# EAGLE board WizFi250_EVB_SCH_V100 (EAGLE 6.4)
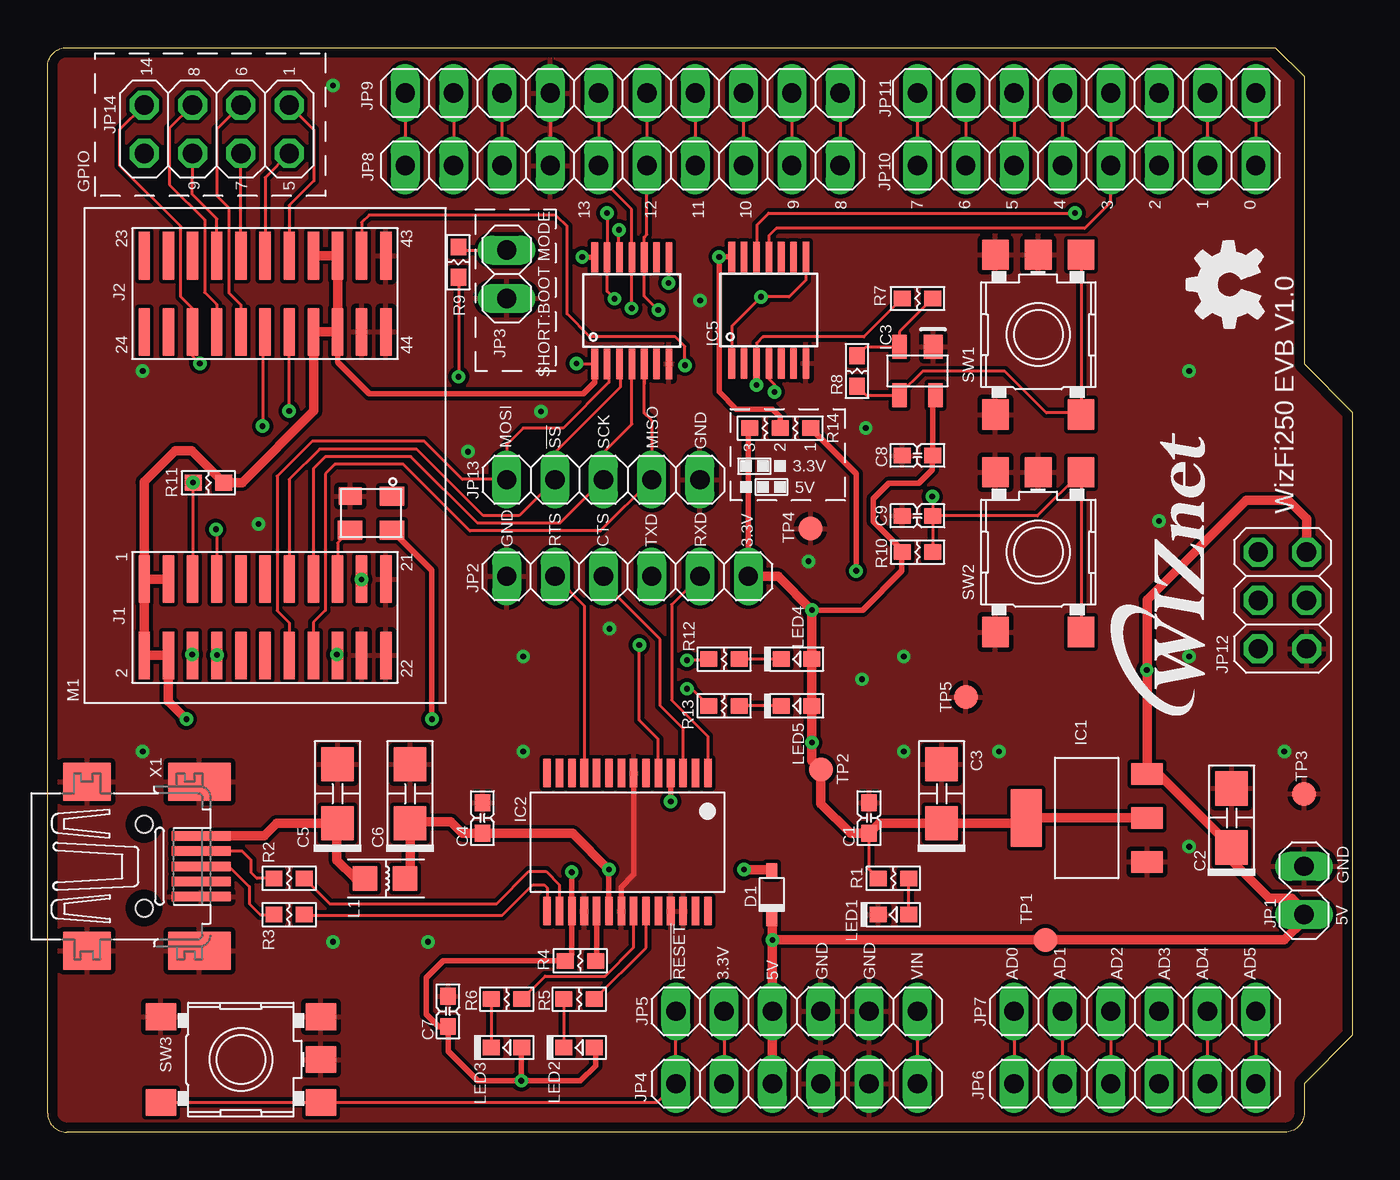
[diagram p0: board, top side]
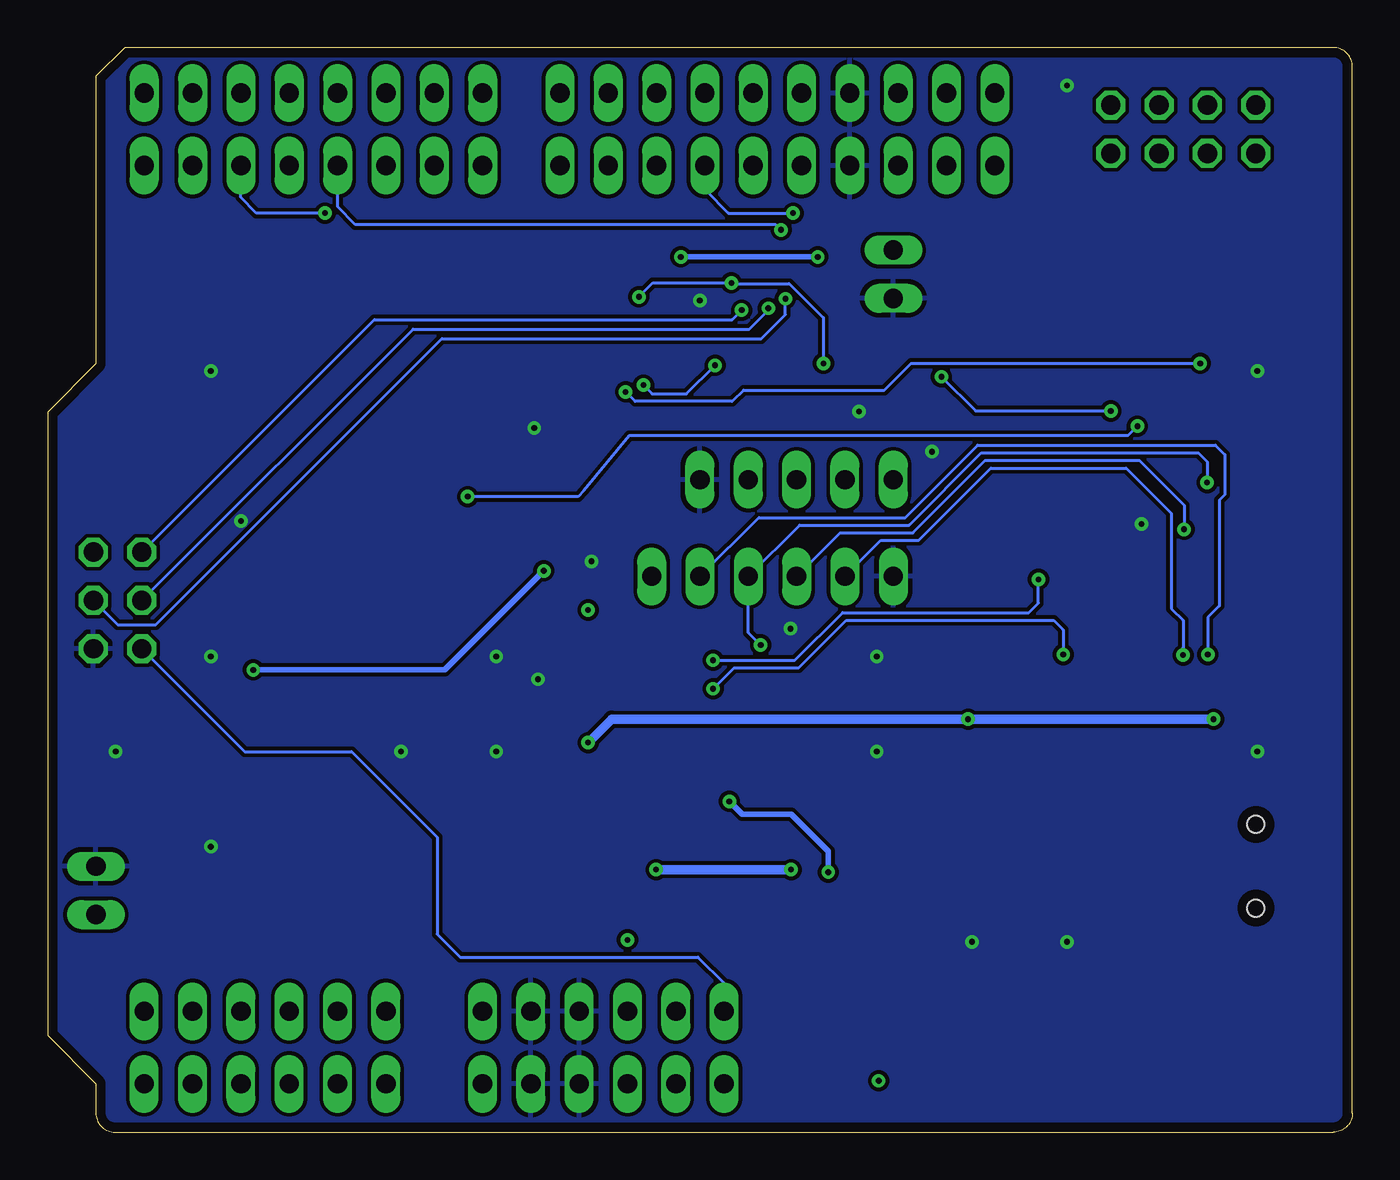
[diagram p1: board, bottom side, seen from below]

Size 68.58 x 57 mm. Coordinates in mm from the lower left corner, seen from the top.
Outline: 0,1 0,56 arc-90 1,57 64.52,57 66.04,55.5 66.04,40.39 68.58,37.85 68.58,5.08 66.04,2.54 66.04,1 arc-90 65.04,0 1,0 arc-90 0,1
Copper layers (1*16): Top 0.035mm / dielectric 1.5mm / Bottom 0.035mm
Design rules "default *": minimum track width 0.1mm, minimum drill 0.2mm, track to track 0.2mm, track to pad 0.2mm, pad to pad 0.2mm, via to via 0.2mm, smd to smd 0.15mm, copper to edge 20mil, drill to drill 0.3mm, minimum pad ring 10mil, minimum via ring 8mil, stop-mask expansion 4mil, vias tented up to drill 12mil, thermal gap 10mil

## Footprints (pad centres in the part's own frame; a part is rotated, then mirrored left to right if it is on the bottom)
C-1608 = smd 0.89 x 0.82: 1 0.8,0; 2 -0.8,0
C-3216(TANTAL) = smd 1.8 x 1.7: 1 1.55,0; 2 -1.55,0
BAT60A = smd 0.8 x 0.6: 1 1.25,0; 2 -1.25,0
SOT-223 = smd 1.143 x 1.651: 1 -2.311,-3.175; 2 0,-3.175; 3 2.311,-3.175 | smd 3 x 1.651: 4 0,3.175
SSOP28 = smd 0.4 x 1.5: 1 -4.225,-3.625; 2 -3.575,-3.625; 3 -2.925,-3.625; 4 -2.275,-3.625; 5 -1.625,-3.625; 6 -0.975,-3.625; 7 -0.325,-3.625; 8 0.325,-3.625; 9 0.975,-3.625; 10 1.625,-3.625; 11 2.275,-3.625; 12 2.925,-3.625; 13 3.575,-3.625; 14 4.225,-3.625; 15 4.225,3.625; 16 3.575,3.625; 17 2.925,3.625; 18 2.275,3.625; 19 1.625,3.625; 20 0.975,3.625; 21 0.325,3.625; 22 -0.325,3.625; 23 -0.975,3.625; 24 -1.625,3.625; 25 -2.275,3.625; 26 -2.925,3.625; 27 -3.575,3.625; 28 -4.225,3.625
MIC811SU = smd 1.016 x 1.27: 1 -0.826,-1.27 | smd 0.762 x 1.27: 2 0.953,-1.27; 3 0.953,1.27; 4 -0.953,1.27
TXS0104EPWR = smd 1.6 x 0.35: 1 -2.8,1.95; 2 -2.8,1.3; 3 -2.8,0.65; 4 -2.8,0; 5 -2.8,-0.65; 6 -2.8,-1.3; 7 -2.8,-1.95; 8 2.8,-1.95; 9 2.8,-1.3; 10 2.8,-0.65; 11 2.8,0; 12 2.8,0.65; 13 2.8,1.3; 14 2.8,1.95
1X02 = drill 1.016 long: 1 -1.27,0; 2 1.27,0
1X06 = drill 1.016 long: 1 -6.35,0; 2 -3.81,0; 3 -1.27,0; 4 1.27,0; 5 3.81,0; 6 6.35,0
1X10 = drill 1.016 long: 1 -11.43,0; 2 -8.89,0; 3 -6.35,0; 4 -3.81,0; 5 -1.27,0; 6 1.27,0; 7 3.81,0; 8 6.35,0; 9 8.89,0; 10 11.43,0
1X08 = drill 1.016 long: 1 -8.89,0; 2 -6.35,0; 3 -3.81,0; 4 -1.27,0; 5 1.27,0; 6 3.81,0; 7 6.35,0; 8 8.89,0
2X03 = drill 1.016 octagon: 1 -2.54,-1.27; 2 -2.54,1.27; 3 0,-1.27; 4 0,1.27; 5 2.54,-1.27; 6 2.54,1.27
1X05 = drill 1.016 long: 1 -5.08,0; 2 -2.54,0; 3 0,0; 4 2.54,0; 5 5.08,0
2X04 = drill 1.016 octagon: 1 -3.81,-1.27; 2 -3.81,1.27; 3 -1.27,-1.27; 4 -1.27,1.27; 5 1.27,-1.27; 6 1.27,1.27; 7 3.81,-1.27; 8 3.81,1.27
L-2012 = smd 1.3 x 1.3: 1 -1.1,0; 2 1,0
LED-1608 = smd 0.89 x 0.82: 1 -0.8,0; 2 0.8,0
WIZFI250-IFBD = smd 2.5 x 0.6: 1 -6.5,6.35; 2 -10.5,6.35; 3 -6.5,5.08; 4 -10.5,5.08; 5 -6.5,3.81; 6 -10.5,3.81; 7 -6.5,2.54; 8 -10.5,2.54; 9 -6.5,1.27; 10 -10.5,1.27; 11 -6.5,0; 12 -10.5,0; 13 -6.5,-1.27; 14 -10.5,-1.27; 15 -6.5,-2.54; 16 -10.5,-2.54; 17 -6.5,-3.81; 18 -10.5,-3.81; 19 -6.5,-5.08; 20 -10.5,-5.08; 21 -6.5,-6.35; 22 -10.5,-6.35; 23 10.5,6.35; 24 6.5,6.35; 25 10.5,5.08; 26 6.5,5.08; 27 10.5,3.81; 28 6.5,3.81; 29 10.5,2.54; 30 6.5,2.54; 31 10.5,1.27; 32 6.5,1.27; 33 10.5,0; 34 6.5,0; 35 10.5,-1.27; 36 6.5,-1.27; 37 10.5,-2.54; 38 6.5,-2.54; 39 10.5,-3.81; 40 6.5,-3.81; 41 10.5,-5.08; 42 6.5,-5.08; 43 10.5,-6.35; 44 6.5,-6.35
R-1608 = smd 0.89 x 0.82: 1 -0.8,0; 2 0.8,0
R-1608-JUMPER = smd 0.89 x 0.82: 1 -1.6,0; 2 0,0; 3 1.6,0
SKHMPXE010 = smd 1.6 x 1.4: 1 -4.2,2.25; 2 4.2,2.25; 3 -4.2,-2.25; 4 4.2,-2.25; 5 4.2,0
B1,27 = smd 1.27 x 1.27: TP 0,0
32005-201 = smd 3.1 x 0.5: 1 3,1.6; 2 3,0.8; 3 3,0; 4 3,-0.8; 5 3,-1.6 | smd 2.5 x 2: M1 -3,-4.45; M2 -3,4.45 | smd 3.3 x 2: M3 2.9,4.45; M4 2.9,-4.45 | hole 0.9: 0,2.2; 0,-2.2
OSC3225 = smd 1.3 x 1: 1 -1.1,-0.9; 3 1.1,0.9; 4 -1.1,0.9 | smd 1.2 x 0.9: 2 1.1,-0.9

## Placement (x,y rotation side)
C1  0.1uF  [C-1608]  43.18,16.51 90 top
C2  10uF/16V  [C-3216(TANTAL)]  62.23,16.51 270 top
C3  10uF/16V  [C-3216(TANTAL)]  46.99,17.78 270 top
C4  0.1uF  [C-1608]  22.86,16.51 90 top
C5  10uF/16V  [C-3216(TANTAL)]  15.24,17.78 270 top
C6  4.7uF/16V  [C-3216(TANTAL)]  19.05,17.78 270 top
C7  0.1uF  [C-1608]  21.05,6.35 90 top
C8  0.1uF  [C-1608]  45.72,35.56 180 top
C9  0.1uF  [C-1608]  45.72,32.38 180 top
D1  BAT60A  [BAT60A]  38.06,12.48 270 top
IC1  AME8815BEGT330  [SOT-223]  54.61,16.51 90 top
IC2  FT232RL  [SSOP28]  30.48,15.24 180 top
IC3  MIC811SU  [MIC811SU]  45.72,40.01 180 top
IC4  TXS0104EPWR  [TXS0104EPWR]  30.71,43.18 90 top
IC5  TXS0104EPWR  [TXS0104EPWR]  37.91,43.2 90 top
JP1  [1X02]  66.04,12.7 90 top
JP2  [1X06]  30.48,29.21 180 top
JP3  [1X02]  24.13,45.09 270 top
JP4  [1X06]  39.37,2.54 0 top
JP5  [1X06]  39.37,6.35 0 top
JP6  [1X06]  57.15,2.54 0 top
JP7  [1X06]  57.15,6.35 0 top
JP8  [1X10]  30.23,50.8 180 top
JP9  [1X10]  30.23,54.61 180 top
JP10  [1X08]  54.61,50.8 180 top
JP11  [1X08]  54.61,54.61 180 top
JP12  [2X03]  64.9,27.94 270 top
JP13  [1X05]  29.21,34.29 0 top
JP14  [2X04]  8.89,52.7 180 top
L1  MI0805K400R-10  [L-2012]  17.78,13.34 0 top
LED1  POWER  [LED-1608]  44.45,11.43 180 top
LED2  RX  [LED-1608]  27.94,4.45 180 top
LED3  TX  [LED-1608]  24.13,4.45 180 top
LED4  Wi-Fi  [LED-1608]  39.37,24.86 180 top
LED5  Mode  [LED-1608]  39.37,22.4 180 top
M1  WIZFI250-IFBD  [WIZFI250-IFBD]  11.43,35.56 90 top
R1  330R  [R-1608]  44.45,13.34 180 top
R2  22R  [R-1608]  12.7,13.34 0 top
R3  22R  [R-1608]  12.7,11.43 0 top
R4  10K  [R-1608]  28,9 0 top
R5  330R  [R-1608]  27.94,6.99 180 top
R6  330R  [R-1608]  24.13,6.99 180 top
R7  1K  [R-1608]  45.72,43.81 180 top
R8  0R  [R-1608]  42.55,40.01 90 top
R9  10K  [R-1608]  21.59,45.72 270 top
R10  10K  [R-1608]  45.72,30.48 180 top
R11  10K  [R-1608]  8.45,34.13 0 top
R12  330R  [R-1608]  35.56,24.86 180 top
R13  330R  [R-1608]  35.56,22.4 0 top
R14  0R-JUMPER  [R-1608-JUMPER]  38.5,37 180 top
SW1  W-RESET  [SKHMPXE010]  52.07,41.91 90 top
SW2  FUNCTION  [SKHMPXE010]  52.07,30.48 90 top
SW3  RESET  [SKHMPXE010]  10.16,3.81 0 top
TP1  TPB1,27  [B1,27]  52.45,10.1 0 top
TP2  TPB1,27  [B1,27]  40.64,19.05 0 top
TP3  TPB1,27  [B1,27]  66.04,17.78 0 top
TP4  TPB1,27  [B1,27]  40.1,31.72 0 top
TP5  TPB1,27  [B1,27]  48.26,22.86 0 top
U$1  [OSHP-LOGO]  64.5,41.5 90 top
U$2  [WIZNET2-LOGO]  62,21 90 top
X1  MINI-USB-SCHIELD-32005-201  [32005-201]  5.08,13.97 0 top
Y1  OSC3225  [OSC3225]  17,32.53 180 top

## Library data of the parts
C1-C9 = CAP
D1 LED1-LED5 = DIODE
IC1 = RECULATOR
IC2 = ftdichip; MPN: FT232RL; OC_FARNELL: 1146032; OC_NEWARK: 91K9918
IC3-IC5 = IC
JP1-JP14 = pinhead
L1 = INDUCTOR
M1 = WIZnet
R1-R14 = RESISTOR
SW1-SW3 = switch
TP1-TP5 = testpad
U$1 U$2 = LOGO
X1 = USB; OC_FARNELL: unknown; OC_NEWARK: unknown
Y1 = X-TAL

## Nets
!RESET: IC5.3 M1.41 R7.2
+3V3: C1.2 C3.1 C8.2 IC1.2 IC1.4 IC3.4 IC4.1 IC4.8 IC5.1 IC5.8 JP2.1 LED4.1 LED5.1 M1.1 M1.2 M1.3 M1.4 M1.37 M1.38 M1.39 M1.40 R1.2 R10.2 R11.2 R14.3 TP2.TP Y1.4
+5V: C2.1 D1.1 IC1.3 JP1.1 JP4.3 JP5.3 JP12.2 R14.1 TP1.TP
BOOT_MODE: M1.36 R9.2
CTS: IC2.3 JP2.4 M1.7
FACTORY_RESET: C9.2 M1.34 R10.1 SW2.3 SW2.4
GND: C1.1 C2.2 C3.2 C4.1 C5.2 C6.2 C7.1 C8.1 C9.1 IC1.1 IC2.7 IC2.18 IC2.21 IC2.25 IC2.26 IC3.1 IC4.7 IC5.7 JP1.2 JP2.6 JP3.2 JP4.4 JP4.5 JP5.4 JP5.5 JP8.7 JP9.7 JP12.6 JP13.5 LED1.2 M1.20 M1.21 M1.22 M1.42 M1.43 M1.44 SW1.1 SW1.2 SW1.5 SW2.1 SW2.2 SW2.5 SW3.1 SW3.2 SW3.5 TP3.TP TP4.TP TP5.TP X1.5 X1.M1 X1.M2 X1.M3 X1.M4 Y1.2
GPIO1: JP14.1 M1.35
GPIO5: JP14.2 M1.33
GPIO6: JP14.3 M1.32
GPIO7: JP14.4 M1.31
GPIO8: JP14.5 M1.30
GPIO9: JP14.6 M1.29
GPIO14: IC5.4 JP14.7 M1.28
MISO: IC4.10 JP8.5 JP9.5 JP12.1
MOSI: IC4.13 JP8.4 JP9.4 JP12.4
N$1: IC4.14 IC5.14 R14.2
N$2: R2.1 X1.2
N$3: R3.1 X1.3
N$4: LED1.1 R1.1
N$5: JP3.1 R9.1
N$6: IC2.16 R2.2
N$7: IC2.15 R3.2
N$8: IC2.19 R4.2
N$9: IC3.2 R7.1 R8.2
N$16: LED2.2 R5.2
N$17: LED3.2 R6.2
N$18: JP4.2 JP5.2
N$22: JP4.6 JP5.6
N$23: JP6.1 JP7.1
N$24: JP6.2 JP7.2
N$25: JP6.3 JP7.3
N$26: JP6.4 JP7.4
N$27: JP6.5 JP7.5
N$28: JP6.6 JP7.6
N$29: JP8.10 JP9.10
N$30: JP8.9 JP9.9
N$31: JP8.8 JP9.8
N$36: JP8.3 JP9.3
N$37: JP8.2 JP9.2
N$38: JP8.1 JP9.1
N$39: JP10.8 JP11.8
N$40: JP10.7 JP11.7
N$41: JP10.6 JP11.6
N$45: JP10.2 JP11.2
N$46: JP10.1 JP11.1
N$50: M1.17 Y1.3
N$51: M1.19 R12.2
N$52: LED4.2 R12.1
N$64: M1.18 R13.1
N$65: LED5.2 R13.2
RESET: JP4.1 JP5.1 JP12.5 SW3.3 SW3.4
RTS: IC2.11 JP2.5 M1.8
RX-LED: IC2.23 R5.1
RXD: IC2.1 JP2.2 M1.6
SCLK: IC4.11 JP8.6 JP9.6 JP12.3
SPI_MISO: IC4.5 JP13.4 M1.16
SPI_MOSI: IC4.2 JP13.1 M1.14
SPI_SCK: IC4.4 JP13.3 M1.15
SPI_SS: IC4.3 JP13.2 M1.13
SS_WIFI: IC4.12 JP10.5 JP11.5
TX-LED: IC2.22 R6.1
TXD: IC2.5 JP2.3 M1.5 R11.1
USB: C4.2 C6.1 D1.2 IC2.20 L1.2
VCC: C5.1 L1.1 X1.1
VCCIO: C7.2 IC2.4 IC2.17 LED2.1 LED3.1 R4.1
W_GPIO14: IC5.11 JP10.4 JP11.4
W_RESET: IC5.12 JP10.3 JP11.3
WI-FI_RST: IC3.3 R8.1 SW1.3 SW1.4

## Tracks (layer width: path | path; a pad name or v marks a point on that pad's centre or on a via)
!RESET  (via drill 0.3)
  Top 0.15: M1.41 16.51,47.81 16.9,48.2 26.7,48.2 27.3,47.6 27.3,43 28.5,41.8 33,41.8 33.5,41.3 v33.5,40.3 | R7.2 42.9,41.8 37.6,41.8 37.26,41.46 IC5.3 | IC5.3 | IC5.3 v37.26,39.26
  Bottom 0.15: v37.26,39.26 36.8,38.8 35,38.8 v33.5,40.3
+3V3  (via drill 0.3)
  Top 0.15: IC4.8 32.64,45.96 v32.64,44.63 | v27.8,40.4 27.82,40.38 IC4.1 | R1.2 43.18,13.8 C1.2 | IC5.8 | IC5.8 39.86,44.78 38.98,43.9 v37.5,43.9 35.96,42.36 IC5.1
  Top 0.3: IC3.4 46.52,38.58 C8.2 46.5,35.54 46.5,34.8 45.8,34.1 44.2,34.1 43.4,33.3 43.4,32.1 44.92,30.58 R10.2 44.9,30.46 44.9,29.5 42.84,27.44 v40.17,27.44 | Y1.4 20.2,29.53 v20.2,21.7 | IC4.1 28.76,39.41 28.15,38.8 16.9,38.8 15.24,40.46 M1.40 | R14.3 36.83,36.93 JP2.1
  Top 0.5: IC1.2 IC1.4 51.16,16.23 C3.1 43.7,16.23 C1.2 42.2,15.7 40.64,17.26 TP2.TP 40.17,19.52 v40.17,20.47 LED5.1 LED4.1 v40.17,27.44 38.4,29.21 JP2.1 | M1.1 M1.2 M1.4 6.35,22.65 v7.3,21.7 | M1.1 M1.3 | M1.37 M1.39 M1.40 M1.38 14,42.03 14,37.9 10.23,34.13 R11.2 7.58,35.8 6.7,35.8 5.08,34.18 M1.1
  Bottom 0.15: v27.8,40.4 27.8,42.8 29.6,44.6 32.61,44.6 v32.64,44.63 36.77,44.63 v37.5,43.9
  Bottom 0.5: v40.17,20.47 38.94,21.7 v20.2,21.7 v7.3,21.7
+5V  (via drill 0.3)
  Top 0.3: v57.77,24.29 57.78,24.3 | R14.1 42.5,34.6 v42.5,29.5
  Top 0.5: JP4.3 JP5.3 v38.1,10.1 | D1.1 38.1,11.19 v38.1,10.1 | v38.1,10.1 TP1.TP 65,10.1 66.04,11.14 JP1.1 65.9,11.57 65.9,11.8 65.4,12.3 64.2,12.3 62.23,14.27 C2.1 58.37,18.82 IC1.3 57.78,24.3 57.78,27.98 63,33.2 65.2,33.2 66.17,32.23 JP12.2
  Bottom 0.3: v42.5,29.5 47.71,24.29 v57.77,24.29
BOOT_MODE  (via drill 0.3)
  Top 0.15: R9.2 v21.6,39.7 | v12.7,37.9 M1.36
  Bottom 0.15: v21.6,39.7 19.8,37.9 v12.7,37.9
CTS  (via drill 0.3)
  Top 0.15: v8.85,31.68 8.89,31.64 M1.7 | IC2.3 33.41,21.21 32.2,22.42 32.2,25.9 29.21,28.89 JP2.4
  Bottom 0.15: JP2.4 26.92,31.5 23.1,31.5 19.3,35.3 11.2,35.3 8.85,32.95 v8.85,31.68
FACTORY_RESET  (via drill 0.3)
  Top 0.15: C9.2 R10.1 | SW2.3 SW2.4 52.02,32.38 C9.2 | M1.34 11.3,41.93 v11.3,37.1 | v46.5,33.4 46.52,33.38 C9.2
  Bottom 0.15: v11.3,37.1 11.8,36.6 38,36.6 40.4,33.7 40.7,33.4 v46.5,33.4
GND  (via drill 0.3)
  Top 0.15: JP9.7 JP8.7
  Top 0.3: IC2.7 30.81,13.55 30.14,12.88 30.14,11.63 IC2.21
  other vias: 65,20 45,20 45,25 25,25 25,20 5,40 5,20 15,10 20,10 40,30 43,37 42.8,23.8 34.3,43.7 60,40 60,25 60,15 50,20 15,55 11.08,31.96 22.1,35.76 25.94,37.87 29.53,26.46 58.41,32.12
  pour Top: 0,0 69,0 69,57 0,57
  pour Bottom: 0,0 69,0 69,57 0,57
GPIO1
  Top 0.15: JP14.1 14,52.67 14,50 12.7,48.7 M1.35
GPIO5
  Top 0.15: JP14.2 11.43,50.16 M1.33
GPIO6
  Top 0.15: JP14.3 8.9,52.72 8.9,49.2 9.53,48.57 9.53,44.11 10.16,43.48 M1.32
GPIO7
  Top 0.15: M1.31 JP14.4
GPIO8
  Top 0.15: JP14.5 6.4,52.76 6.4,49.8 8.26,47.94 8.26,44.13 8.89,43.5 M1.30
GPIO9
  Top 0.15: M1.29 8.9,48 7.6,49.3 7.6,50.1 7.62,50.12 JP14.6
GPIO14  (via drill 0.3)
  Top 0.15: JP14.7 3.8,52.7 3.8,50.8 7,47.6 7,47.58 6.99,47.57 6.99,43.91 7.6,43.3 7.6,42.08 M1.28 7.62,40.78 v8,40.4 | IC5.4 37.9,39.6 38.2,39.3 v38.2,38.9
  Bottom 0.15: v8,40.4 23.2,40.4 24.6,39 32,39 32.6,38.4 37.7,38.4 v38.2,38.9
MISO  (via drill 0.3)
  Top 0.15: JP9.5 JP8.5 31.5,47.19 31.35,47.04 IC4.10 31.36,43.94 v32.1,43.2
  Bottom 0.15: JP12.1 51.41,42.7 32.6,42.7 v32.1,43.2
MOSI  (via drill 0.3)
  Top 0.15: JP9.4 JP8.4 | IC4.13 | v29.8,43.8 29.41,44.19 IC4.13 | v29.4,48.3 v29.41,48.29 IC4.13
  Bottom 0.15: JP12.4 64.9,26.67 62.89,26.67 47.86,41.7 31.06,41.7 29.8,42.96 v29.8,43.8 | JP8.4 34,50.76 34,49.5 32.8,48.3 v29.4,48.3
N$1  (via drill 0.3)
  Top 0.3: IC5.14 | IC5.14 v35.3,46 35.3,38.9 36.2,38 38.1,38 38.5,37.6 R14.2 | v28.1,46 28.12,45.98 IC4.14 | R14.2
  Bottom 0.3: v35.3,46 v28.1,46
N$2
  Top 0.15: R2.1 11,13.34 10.7,13.64 10.7,14.3 10.23,14.77 X1.2
N$3
  Top 0.15: X1.3 8.15,13.9 9.6,13.9 10.6,12.9 10.6,12 11.17,11.43 R3.1
N$4
  Top 0.15: LED1.1 R1.1
N$5
  Top 0.15: R9.1 21.75,46.35 JP3.1
N$6
  Top 0.15: R2.2 14.84,12 23.6,12 25.3,13.7 26.2,13.7 26.91,12.99 IC2.16
N$7
  Top 0.15: R3.2 13.53,11.4 23.9,11.4 25.5,13 26.1,13 26.25,12.85 IC2.15
N$8
  Top 0.3: R4.2 28.86,9.05 IC2.19
N$9
  Top 0.15: R7.1 44.77,42.06 IC3.2 43.02,41.27 R8.2
N$16
  Top 0.15: R5.2 LED2.2
N$17
  Top 0.15: R6.2 LED3.2
N$18
  Top 0.15: JP5.2 JP4.2
N$22
  Top 0.15: JP5.6 JP4.6
N$23
  Top 0.15: JP7.1 JP6.1
N$24
  Top 0.15: JP7.2 JP6.2
N$25
  Top 0.15: JP7.3 JP6.3
N$26
  Top 0.15: JP7.4 JP6.4
N$27
  Top 0.15: JP7.5 JP6.5
N$28
  Top 0.15: JP7.6 JP6.6
N$29
  Top 0.15: JP9.10 JP8.10
N$30
  Top 0.15: JP9.9 JP8.9
N$31
  Top 0.15: JP9.8 JP8.8
N$36
  Top 0.15: JP9.3 JP8.3
N$37
  Top 0.15: JP9.2 JP8.2
N$38
  Top 0.15: JP9.1 JP8.1
N$39
  Top 0.15: JP11.8 JP10.8
N$40
  Top 0.15: JP11.7 JP10.7
N$41
  Top 0.15: JP11.6 JP10.6
N$45
  Top 0.15: JP11.2 JP10.2
N$46
  Top 0.15: JP11.1 JP10.1
N$50
  Top 0.15: Y1.3 15.24,30.97 M1.17
N$51  (via drill 0.3)
  Top 0.15: R12.2 34.7,24.8 v33.6,24.8 | M1.19 v16.5,29.05
  Bottom 0.15: v33.6,24.8 29.3,24.8 26.8,27.3 17,27.3 16.5,27.8 v16.5,29.05
N$52
  Top 0.15: LED4.2 R12.1
N$64  (via drill 0.3)
  Top 0.15: R13.1 33.86,23.3 v33.6,23.3 | M1.18 v15.2,25.1
  Bottom 0.15: v33.6,23.3 32.5,24.4 29.1,24.4 26.6,26.9 15.7,26.9 15.2,26.4 v15.2,25.1
N$65
  Top 0.15: LED5.2 R13.2
RESET
  Top 0.15: JP5.1 JP4.1 32.04,1.56 SW3.4 SW3.3
  Bottom 0.15: JP12.5 58.23,20 52.6,20 48.1,15.5 48.1,10.4 46.9,9.2 34.4,9.2 33.02,7.82 JP5.1 33.02,5.8
RTS  (via drill 0.3)
  Top 0.15: M1.8 v8.9,25.07 | JP2.5 28.2,27.68 IC2.11
  Bottom 0.15: JP2.5 24.78,31.1 22.8,31.1 19,34.9 11.9,34.9 9.52,32.52 9.52,27.51 8.9,26.89 v8.9,25.07 8.9,25.47
RX-LED
  Top 0.15: R5.1 31.45,9.7 IC2.23
RXD  (via drill 0.3)
  Top 0.15: M1.6 7.5,25.18 v7.6,25.1 | JP2.2 32.8,27.72 32.8,22.7 34.7,20.8 IC2.1
  Bottom 0.15: JP2.2 31.2,32.3 23.5,32.3 19.7,36.1 7.2,36.1 6.7,35.6 6.7,33.5 6.99,33.21 6.99,27.66 7.6,27.05 v7.6,25.1
SCLK  (via drill 0.3)
  Top 0.15: JP9.6 JP8.6 28.96,50.24 30.7,48.5 IC4.11 v30.71,43.31 v30.7,43.3
  Bottom 0.15: JP12.3 49.37,42.2 31.7,42.2 30.7,43.2 v30.7,43.3
SPI_MISO
  Top 0.15: 31.35,39.3 IC4.5 31.36,37.79 31.75,37.4 JP13.4 29.06,31.6 22.2,31.6 18.7,35.1 15.1,35.1 14.6,34.6 14.6,27.42 13.97,26.79 M1.16
SPI_MOSI
  Top 0.15: IC4.2 29.5,40.29 29.5,39.4 27.1,37 25,37 24.13,36.13 JP13.1 | 24.13,35.53 JP13.1 | JP13.1 21.8,34.3 19.8,36.3 13.9,36.3 12.07,34.47 12.07,27.41 12.7,26.78 M1.14
SPI_SCK
  Top 0.15: M1.15 13.97,34.87 14.6,35.5 19.1,35.5 22.6,32 26.92,32 JP13.3 29.22,35.72 30.71,37.21 IC4.4
SPI_SS
  Top 0.15: IC4.3 30.1,40.34 30.1,39.15 26.69,35.74 26.69,34.31 JP13.2 24.78,32.4 22.9,32.4 19.4,35.9 14.3,35.9 12.7,34.3 M1.13
SS_WIFI  (via drill 0.3)
  Top 0.15: JP11.5 JP10.5 | IC4.12 30.03,46.01 v30.03,47.42
  Bottom 0.15: v30.03,47.42 30.31,47.7 52.4,47.7 53.34,48.64 JP10.5
TX-LED
  Top 0.15: R6.1 26.14,8.2 29.3,8.2 30.8,9.71 IC2.22
TXD  (via drill 0.3)
  Top 0.15: 7.61,34.17 v7.64,34.14 R11.1 7.62,34.1 M1.5 | IC2.5 32.09,18.88 32.09,20.66 31.1,21.65 v31.1,25.6
  Bottom 0.15: v7.64,34.14 7.64,35.24 8.1,35.7 19.5,35.7 23.3,31.9 29.06,31.9 JP2.3 31.75,26.25 v31.1,25.6
USB  (via drill 0.3)
  Top 0.3: v29.5,13.8 v29.5,13.79 IC2.20
  Top 0.5: L1.2 19.05,13.61 C6.1 19.12,16.3 21.2,16.3 21.79,15.71 C4.2 27.6,15.7 v29.5,13.8 | D1.2 37.99,13.8 v36.6,13.8
  Bottom 0.5: v29.5,13.8 v36.6,13.8
VCC
  Top 0.5: X1.1 11.38,15.57 12.04,16.23 C5.1 15.2,16.19 15.2,14.3 16.16,13.34 L1.1
VCCIO  (via drill 0.3)
  Top 0.3: LED2.1 28.8,4.38 28.8,3.5 28,2.7 v24.9,2.7 | v24.9,2.7 22.6,2.7 21.05,4.25 C7.2 20.55,5.55 19.9,6.2 19.9,8.1 20.8,9 R4.1 27.55,9.36 IC2.17 v27.55,13.65 v27.55,13.66 | LED3.1 24.9,4.42 v24.9,2.7 | IC2.4 v32.75,17.38
  Bottom 0.3: v32.75,17.38 32.07,16.7 29.5,16.7 27.55,14.75 v27.55,13.66
W_GPIO14
  Top 0.15: JP11.4 JP10.4 55.88,48.88 54.5,47.5 38.3,47.5 37.91,47.11 IC5.11
W_RESET  (via drill 0.3)
  Top 0.15: JP11.3 JP10.3 | IC5.12 37.3,46.04 37.3,47.7 37.9,48.3 v54,48.3
  Bottom 0.15: v54,48.3 57.6,48.3 58.42,49.12 JP10.3
WI-FI_RST
  Top 0.15: SW1.4 SW1.3 54.23,37.8 52.5,37.8 50.3,40 46,40 44.77,38.77 IC3.3 43.02,38.73 R8.1

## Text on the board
tPlace: 14 | 8 | 6 | 1 | GPIO | 9 | 7 | 5 | SHORT:BOOT MODE | 13 | 12 | 11 | 10 | 9 | 8 | 7 | 6 | 5 | 4 | 3 | 2 | 1 | 0 | MOSI | !SS | SCK | MISO | GND | 3 | 2 | 1 | 3.3V | 5V | WizFi250 EVB V1.0 | GND | RTS | CTS | TXD | RXD | 3.3V | GND | 5V | !RESET | 3.3V | 5V | GND | GND | VIN | AD0 | AD1 | AD2 | AD3 | AD4 | AD5
tValues: GND | GND | 3.3V | GND | 5V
